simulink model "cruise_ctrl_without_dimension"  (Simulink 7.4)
settings: Solver=ode45  StartTime=0.0  StopTime=30  MaxStep=0.1  RelTol=1e-3
PreLoadFcn:
  | m = 1000;
  | alpha = [40, 25, 16, 12, 10];
  | Tm = 190;
  | wm = 420;
  | beta = 0.4;
  | Cr = 0.01;
  | rho = 1.3;
  | Cd = 0.32;
  | A = 2.4;
  | g = 9.8;
  | theta = 0;
  | gear = 3;
libraries: simulink x1

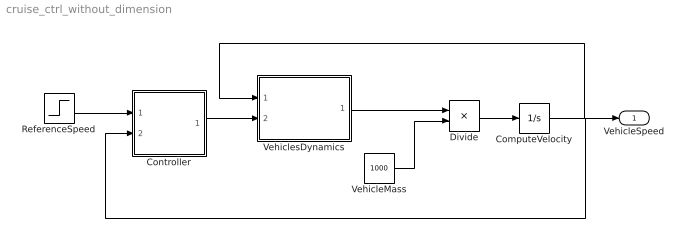
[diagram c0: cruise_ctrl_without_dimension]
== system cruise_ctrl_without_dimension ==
  ComputeVelocity : Integrator  InitialCondition=20
  Controller : Subsystem  Description=|
      | begin dimension     
      | (assert (= In1 In2))
      | end dimension
  Divide : Product  Inputs=*/  OutDataType=fixdt(1, 16)  OutScaling=2^-10
  ReferenceSpeed : Step  Time=0  After=30  SampleTime=0
  VehicleMass : Constant  Value=1000  OutDataType=fixdt(1, 16)  OutScaling=2^0
  VehiclesDynamics : Subsystem
  VehicleSpeed : Outport  OutDataType=fixdt(1, 16)  OutScaling=2^0
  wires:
  ComputeVelocity/1 -> VehiclesDynamics/1(In1), VehicleSpeed/1, Controller/2(In2)
  Controller/1(Out1) -> VehiclesDynamics/2(In2)
  ReferenceSpeed/1 -> Controller/1(In1)
  VehiclesDynamics/1(Out1) -> Divide/1
  VehicleMass/1 -> Divide/2
  Divide/1 -> ComputeVelocity/1

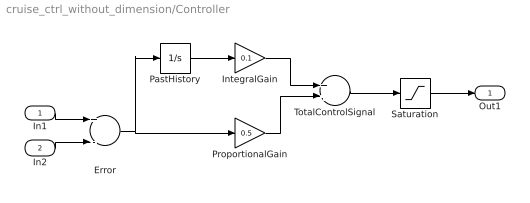
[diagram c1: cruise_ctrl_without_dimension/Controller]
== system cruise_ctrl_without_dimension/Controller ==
  In1 : Inport
  In2 : Inport  Port=2
  Error : Sum  Inputs=+-  OutDataType=sfix(16)  OutScaling=2^-10
  IntegralGain : Gain  Gain=0.1  ParameterDataType=sfix(16)  ParameterScaling=2^0  OutDataType=sfix(16)  OutScaling=2^0
  PastHistory : Integrator  InitialCondition=0.9
  ProportionalGain : Gain  Gain=0.5  ParameterDataType=sfix(16)  ParameterScaling=2^0  OutDataType=sfix(16)  OutScaling=2^0
  Saturation : Saturate  UpperLimit=1  LowerLimit=0
  TotalControlSignal : Sum  OutDataType=sfix(16)  OutScaling=2^-10
  Out1 : Outport  Description=|
      | begin dimension      
      | input _ : [(dimensionless)];
      | end dimension
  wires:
  TotalControlSignal/1 -> Saturation/1
  ProportionalGain/1 -> TotalControlSignal/2
  IntegralGain/1 -> TotalControlSignal/1
  Error/1 -> ProportionalGain/1, PastHistory/1
  PastHistory/1 -> IntegralGain/1
  In2/1 -> Error/2
  Saturation/1 -> Out1/1
  In1/1 -> Error/1

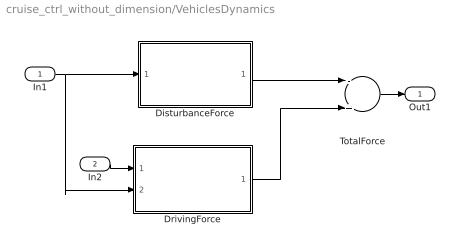
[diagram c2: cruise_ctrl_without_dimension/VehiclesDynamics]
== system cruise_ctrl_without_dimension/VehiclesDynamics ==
  In1 : Inport  Description=|
      | begin dimension                               
      | output _ : [(length metre 1, time second -1)];
      | end dimension
  In2 : Inport  Description=|  Port=2
      | begin dimension       
      | output _ : [(dimensionless)];
      | end dimension
  DisturbanceForce : Subsystem
  DrivingForce : Subsystem
  TotalForce : Sum  Inputs=-+  OutDataType=sfix(16)  OutScaling=2^-10
  Out1 : Outport  Description=|
      | begin dimension                                               
      | input _ : [(length metre 1, mass kilogram 1, time second -2)];
      | end dimension
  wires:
  DrivingForce/1(Out1) -> TotalForce/2
  DisturbanceForce/1(Out1) -> TotalForce/1
  In1/1 -> DisturbanceForce/1(In1), DrivingForce/2(In2)
  TotalForce/1 -> Out1/1
  In2/1 -> DrivingForce/1(In1)

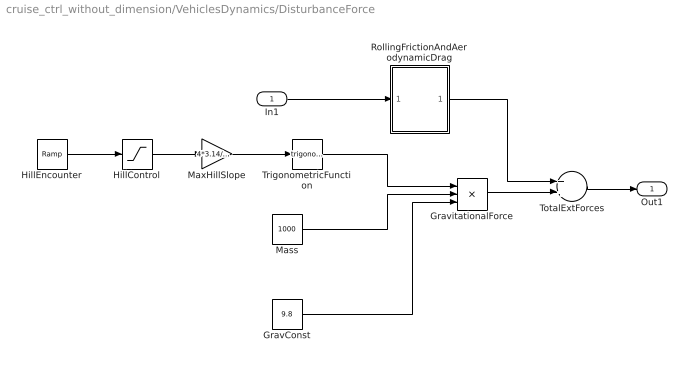
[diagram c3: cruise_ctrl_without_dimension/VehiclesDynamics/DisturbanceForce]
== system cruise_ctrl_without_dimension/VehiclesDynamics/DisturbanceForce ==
  In1 : Inport  Description=|
      | begin dimension                               
      | output _ : [(length metre 1, time second -1)];
      | end dimension
  GravConst : Constant  Description=|  Value=9.8  OutDataType=sfix(16)  OutScaling=2^0
      | begin dimension                               
      | output _ : [(length metre 1, time second -2)];
      | end dimension
  GravitationalForce : Product  Inputs=3  OutDataType=sfix(16)  OutScaling=2^0
  HillControl : Saturate  UpperLimit=1  LowerLimit=0
  HillEncounter : simulink/Sources/Ramp  Description=|  SystemSampleTime=-1  slope=1  start=0  X0=0
      | begin dimension       
      | output 1 : [(dimensionless)];
      | end dimension
  Mass : Constant  Description=|  Value=1000  OutDataType=sfix(16)  OutScaling=2^0
      | begin dimension                
      | output _ : [(mass kilogram 1)];
      | end dimension
  MaxHillSlope : Gain  Description=|  Gain=4*3.14/180  ParameterDataType=sfix(16)  ParameterScaling=2^0  OutDataType=sfix(16)  OutScaling=2^0
      | begin dimension                 
      | constant _ : [(angle radian 1)];
      | end dimension
  RollingFrictionAndAerodynamicDrag : Subsystem
  TotalExtForces : Sum  OutDataType=sfix(16)  OutScaling=2^-10
  TrigonometricFunction : Trigonometry
  Out1 : Outport  Description=|
      | begin dimension                                               
      | input _ : [(length metre 1, mass kilogram 1, time second -2)];
      | end dimension
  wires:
  GravitationalForce/1 -> TotalExtForces/2
  TrigonometricFunction/1 -> GravitationalForce/1
  MaxHillSlope/1 -> TrigonometricFunction/1
  Mass/1 -> GravitationalForce/2
  HillControl/1 -> MaxHillSlope/1
  HillEncounter/1 -> HillControl/1
  TotalExtForces/1 -> Out1/1
  RollingFrictionAndAerodynamicDrag/1(Out2) -> TotalExtForces/1
  In1/1 -> RollingFrictionAndAerodynamicDrag/1(In2)
  GravConst/1 -> GravitationalForce/3

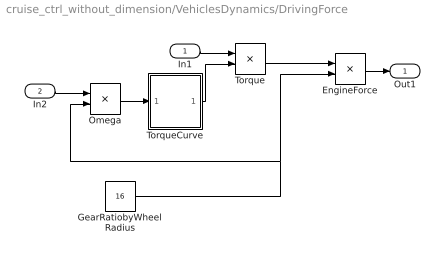
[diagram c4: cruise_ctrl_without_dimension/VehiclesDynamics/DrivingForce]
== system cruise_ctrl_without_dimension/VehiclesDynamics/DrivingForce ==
  In1 : Inport  Description=|
      | begin dimension       
      | output _ : [(dimensionless)];
      | end dimension
  In2 : Inport  Description=|  Port=2
      | begin dimension                               
      | output _ : [(length metre 1, time second -1)];
      | end dimension
  EngineForce : Product  Inputs=**  OutDataType=sfix(16)  OutScaling=2^-10
  GearRatiobyWheelRadius : Constant  Description=|  Value=16  OutDataType=sfix(16)  OutScaling=2^0
      | begin dimension                                
      | output _ : [(length metre -1, angle radian 1)];
      | end dimension
  Omega : Product  OutDataType=sfix(16)  OutScaling=2^0
  Torque : Product  OutDataType=sfix(16)  OutScaling=2^0
  TorqueCurve : Subsystem
  Out1 : Outport  Description=|
      | begin dimension                                               
      | input _ : [(length metre 1, mass kilogram 1, time second -2)];
      | end dimension
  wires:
  GearRatiobyWheelRadius/1 -> EngineForce/2, Omega/2
  Omega/1 -> TorqueCurve/1(In3)
  Torque/1 -> EngineForce/1
  TorqueCurve/1(Out1) -> Torque/2
  In1/1 -> Torque/1
  In2/1 -> Omega/1
  EngineForce/1 -> Out1/1

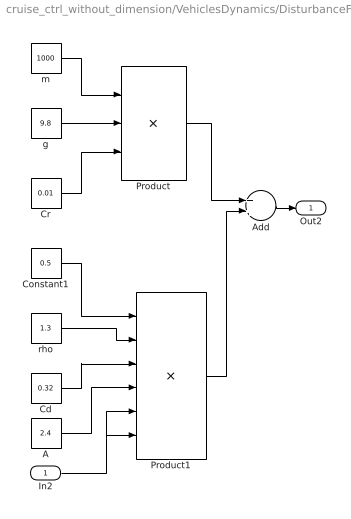
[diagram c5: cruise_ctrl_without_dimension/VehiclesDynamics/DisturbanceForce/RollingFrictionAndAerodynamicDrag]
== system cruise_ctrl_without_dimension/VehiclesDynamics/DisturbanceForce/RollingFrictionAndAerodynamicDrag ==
  In2 : Inport  Description=|
      | begin dimension                               
      | output _ : [(length metre 1, time second -1)];
      | end dimension
  A : Constant  Description=|  Value=2.4  OutDataType=fixdt(1, 16)  OutScaling=2^0
      | begin dimension               
      | output _ : [(length metre 2)];
      | end dimension
  Add : Sum  OutDataType=fixdt(1, 16)  OutScaling=2^-10
  Cd : Constant  Description=|  Value=0.32  OutDataType=fixdt(1, 16)  OutScaling=2^0
      | begin dimension       
      | output _ : [(dimensionless)];
      | end dimension
  Constant1 : Constant  Description=|  Value=0.5  OutDataType=fixdt(1, 16)  OutScaling=2^0
      | begin dimension       
      | output _ : [(dimensionless)];
      | end dimension
  Cr : Constant  Description=|  Value=0.01  OutDataType=fixdt(1, 16)  OutScaling=2^0
      | begin dimension       
      | output _ : [(dimensionless)];
      | end dimension
  Product : Product  Inputs=3  OutDataType=fixdt(1, 16)  OutScaling=2^0
  Product1 : Product  Inputs=6  OutDataType=fixdt(1, 16)  OutScaling=2^0
  g : Constant  Description=|  Value=9.8  OutDataType=fixdt(1, 16)  OutScaling=2^0
      | begin dimension                               
      | output _ : [(length metre 1, time second -2)];
      | end dimension
  m : Constant  Description=|  Value=1000  OutDataType=fixdt(1, 16)  OutScaling=2^0
      | begin dimension                
      | output _ : [(mass kilogram 1)];
      | end dimension
  rho : Constant  Description=|  Value=1.3  OutDataType=fixdt(1, 16)  OutScaling=2^0
      | begin dimension                                 
      | output _ : [(length metre -3, mass kilogram 1)];
      | end dimension
  Out2 : Outport  Description=|
      | begin dimension                                               
      | input _ : [(length metre 1, mass kilogram 1, time second -2)];
      | end dimension
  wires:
  m/1 -> Product/1
  g/1 -> Product/2
  Cr/1 -> Product/3
  Constant1/1 -> Product1/1
  rho/1 -> Product1/2
  Cd/1 -> Product1/3
  A/1 -> Product1/4
  Product/1 -> Add/1
  Product1/1 -> Add/2
  In2/1 -> Product1/5, Product1/6
  Add/1 -> Out2/1

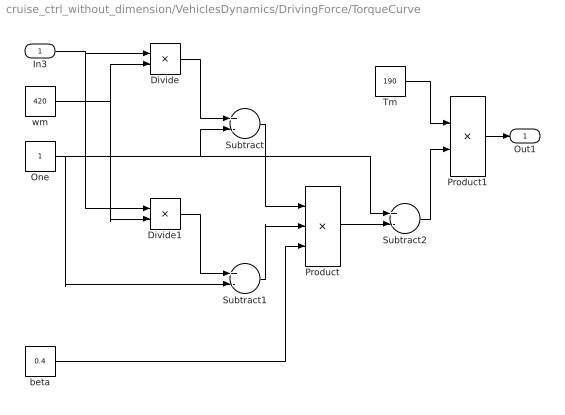
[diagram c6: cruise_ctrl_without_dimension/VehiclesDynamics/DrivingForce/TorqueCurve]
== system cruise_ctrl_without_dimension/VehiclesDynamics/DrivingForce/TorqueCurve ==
  In3 : Inport  Description=|
      | begin dimension                               
      | output _ : [(time second -1, angle radian 1)];
      | end dimension
  Divide : Product  Inputs=*/  OutDataType=fixdt(1, 16)  OutScaling=2^-10
  Divide1 : Product  Inputs=*/  OutDataType=fixdt(1, 16)  OutScaling=2^-10
  One : Constant  Description=|  OutDataType=sfix(16)  OutScaling=2^0
      | begin dimension       
      | output _ : [(dimensionless)];
      | end dimension
  Product : Product  Inputs=3  OutDataType=fixdt(1, 16)  OutScaling=2^0
  Product1 : Product  OutDataType=fixdt(1, 16)  OutScaling=2^0
  Subtract : Sum  Inputs=+-  OutDataType=fixdt(1, 16)  OutScaling=2^-10
  Subtract1 : Sum  Inputs=+-  OutDataType=fixdt(1, 16)  OutScaling=2^-10
  Subtract2 : Sum  Inputs=+-  OutDataType=fixdt(1, 16)  OutScaling=2^-10
  Tm : Constant  Description=|  Value=190  OutDataType=sfix(16)  OutScaling=2^0
      | begin dimension                                                                 
      | output _ : [(length metre 2, mass kilogram 1, time second -2, angle radian -1)];
      | end dimension
  beta : Constant  Description=|  Value=0.4  OutDataType=sfix(16)  OutScaling=2^0
      | begin dimension       
      | output _ : [(dimensionless)];
      | end dimension
  wm : Constant  Description=|  Value=420  OutDataType=sfix(16)  OutScaling=2^0
      | begin dimension                               
      | output _ : [(time second -1, angle radian 1)];
      | end dimension
  Out1 : Outport  Description=|
      | begin dimension                                                                 
      | output _ : [(length metre 2, mass kilogram 1, time second -2, angle radian -1)];
      | end dimension
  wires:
  In3/1 -> Divide/1, Divide1/1
  wm/1 -> Divide/2, Divide1/2
  Divide/1 -> Subtract/1
  One/1 -> Subtract/2, Subtract2/1, Subtract1/2
  Divide1/1 -> Subtract1/1
  Subtract/1 -> Product/1
  Subtract1/1 -> Product/2
  beta/1 -> Product/3
  Product/1 -> Subtract2/2
  Tm/1 -> Product1/1
  Subtract2/1 -> Product1/2
  Product1/1 -> Out1/1
